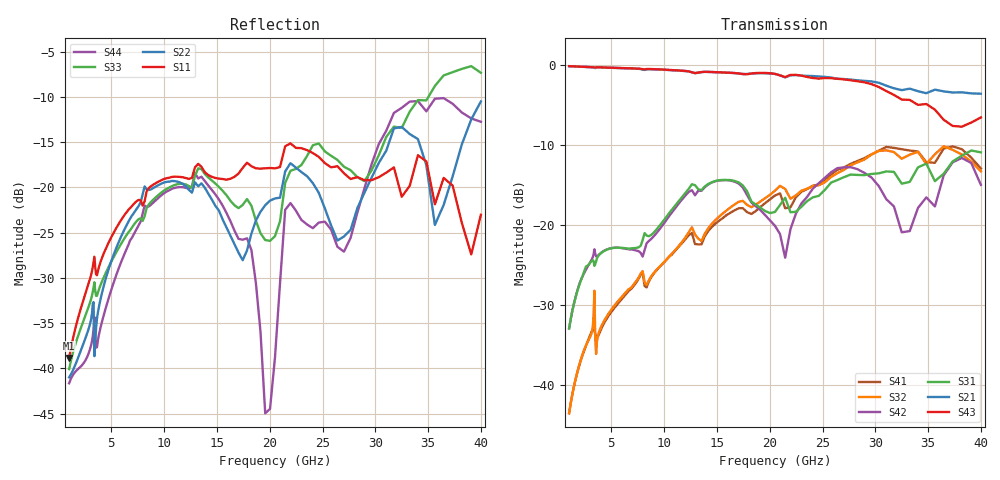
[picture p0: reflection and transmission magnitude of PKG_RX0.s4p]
! Created Mon Sep 18 16:21:07 2017
# hz S ma R 50
! 4 Port Network Data from SP1.SP block
! freq  magS11  angS11  magS12  angS12  magS13  angS13  magS14  angS14
!  magS21  angS21  magS22  angS22  magS23  angS23  magS24  angS24
!  magS31  angS31  magS32  angS32  magS33  angS33  magS34  angS34
!  magS41  angS41  magS42  angS42  magS43  angS43  magS44  angS44
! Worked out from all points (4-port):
!   161 points, 1 GHz to 40 GHz, reference 50 ohm
!   strongest paths, dB at 1 GHz, 2.515 GHz, 6.325 GHz, 15.91 GHz, 40 GHz:
!     S43: -0.1, -0.2, -0.3, -0.9, -6.5
!     S21: -0.1, -0.2, -0.4, -0.9, -3.5
!     S31: -32.9, -25.4, -22.9, -14.3, -10.9
!     S42: -32.9, -25.7, -22.9, -14.3, -14.9
!     S32: -43.5, -35.3, -28.5, -18.1, -13.2
!     S41: -43.5, -35.3, -28.7, -18.7, -12.9
!   lowest |S11| = -38.8 dB at 1 GHz (marker M1), VSWR 1.02, Z = 51.1 + j0.333 ohm
!   |S11| at or under -10 dB: start of sweep to end of sweep
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1e9  0.01142 16.6  0.989 -17.4  0.02269 75.4  0.006682 -111.2
     0.989 -17.4  0.008914 39.7  0.006704 -111.1  0.0227 67.5
     0.02269 75.4  0.006704 -111.1  0.009892 15.6  0.9894 -16.7
     0.006682 -111.2  0.0227 67.5  0.9894 -16.7  0.008265 32.9
5.507478e9  0.06023 -65.8  0.9636 -93.8  0.07255 34.1  0.03173 -179.5
            0.9636 -93.8  0.04691 35.5  0.03282 176.4  0.07255 -36.7
            0.07255 34.1  0.03282 176.4  0.04422 -60.8  0.9655 -90.2
            0.03173 -179.5  0.07255 -36.7  0.9655 -90.2  0.03329 27.6
1.0503e10  0.1131 -111.4  0.9352 -178.3  0.1199 39.6  0.06397 107.0
           0.9352 -178.3  0.1076 -65.0  0.06418 100.9  0.115 152.1
           0.1199 39.6  0.06418 100.9  0.09995 -106.4  0.9377 -171.8
           0.06397 107.0  0.115 152.1  0.9377 -171.8  0.09654 -58.2
1.957316e10  0.1275 -139.0  0.8935 28.9  0.1229 -32.0  0.1378 -49.1
             0.8935 28.9  0.07969 15.5  0.148 -64.5  0.1159 -72.6
             0.1229 -32.0  0.148 -64.5  0.05116 -142.2  0.8975 40.3
             0.1378 -49.1  0.1159 -72.6  0.8975 40.3  0.005639 111.4
2.19647e10  0.1751 -146.2  0.8671 -11.0  0.1208 -37.5  0.1297 -87.4
            0.8671 -11.0  0.1361 -39.8  0.1468 -114.8  0.09476 -159.3
            0.1208 -37.5  0.1468 -114.8  0.1236 -116.7  0.8723 1.1
            0.1297 -87.4  0.09476 -159.3  0.8723 1.1  0.08192 -54.7
3.103976e10  0.1207 -166.7  0.747 -172.1  0.2174 -160.4  0.3093 98.5
             0.747 -172.1  0.1597 -75.7  0.2945 73.3  0.1458 -26.7
             0.2174 -160.4  0.2945 73.3  0.1902 -162.7  0.6915 -159.9
             0.3093 98.5  0.1458 -26.7  0.6915 -159.9  0.2059 -71.5
4e10  0.0706 -73.2  0.6656 34.0  0.2862 46.6  0.2269 -93.2
      0.6656 34.0  0.2986 -26.2  0.2176 -116.2  0.1792 -0.9
      0.2862 46.6  0.2176 -116.2  0.4301 55.1  0.473 70.1
      0.2269 -93.2  0.1792 -0.9  0.473 70.1  0.2306 21.8
